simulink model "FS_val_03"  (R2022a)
settings: Solver=VariableStepAuto  StartTime=0.0  StopTime=300  RelTol=1e-3
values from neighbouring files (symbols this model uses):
  C = 6.3000e-04    (= 0.00063)    [maglev_init.m]
  g = 9.80    (= 9.8)    [maglev_init.m]
  K = 1.0e+03 * [-2.4567   -0.1235    0.0237]    [maglev_init.m]
  L1 = 0.6000    (= 0.6)    [maglev_init.m]
  m = 0.0300    (= 0.03)    [maglev_init.m]
  mpert = 0    [maglev_init.m]
  R = 45    [maglev_init.m]
  Ts = 0.005    [maglev_init.m]    (also in train_net.m)
  x1_0 = 0.1    [maglev_init.m]
  x1_d = 0.05    [maglev_init.m]
  x2_0 = 0    [maglev_init.m]
  x2_d = 0    [maglev_init.m]
  x3_0 = 0.2    [maglev_init.m]
undefined symbols (not defined in the file or in its folder): magnitude
libraries: fuzblock x1

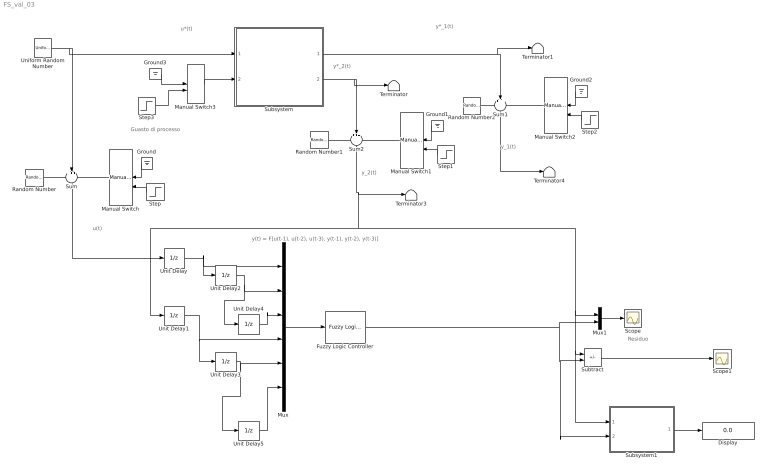
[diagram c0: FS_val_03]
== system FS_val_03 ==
  note: y(t) = F[u(t-1), u(t-2), u(t-3), y(t-1), y(t-2), y(t-3)]
  note: y_2(t)
  note: y*_1(t)
  note: u(t)
  note: y*_2(t)
  note: y_1(t)
  note: u*(t)
  note: Guasto di processo
  note: Residuo
  Display : Display
  Fuzzy Logic Controller : fuzblock/Fuzzy Logic  Controller  FIS=FIS03  OutputSampleNumber=101  DataType=double  FuzzifiedInputs=off  RuleFiringStrengths=off  RuleOutputs=off  AggregatedOutputs=off  SimulateUsing=Interpreted execution  OutOfRangeInputValueMessage=warning  NoRuleFiredMessage=warning  EmptyOutputFuzzySetMessage=warning
  Ground{,1..3} (4 alike) : Ground
  Manual Switch : ManualSwitch
  Manual Switch1 : ManualSwitch  CurrentSetting=0
  Manual Switch2 : ManualSwitch
  Manual Switch3 : ManualSwitch
  Mux : Mux  Inputs=6
  Mux1 : Mux  Inputs=2
  Random Number : RandomNumber  Variance=1e-9  Seed=1  SampleTime=Ts
  Random Number1 : RandomNumber  Variance=1e-6  Seed=3  SampleTime=Ts
  Random Number2 : RandomNumber  Variance=1e-9  Seed=2  SampleTime=Ts
  Scope : Scope
  Scope1 : Scope
  Step : Step  Time=150  SampleTime=0
  Step1 : Step  Time=150  SampleTime=0
  Step2 : Step  Time=150  SampleTime=0
  Step3 : Step  Time=15  After=2*R  SampleTime=0
  Subsystem : Subsystem
  Subsystem1 : Subsystem
  Subtract : Sum  Inputs=+-
  Sum : Sum  Inputs=+++
  Sum1 : Sum  Inputs=+++
  Sum2 : Sum  Inputs=+++
  Terminator{,1,3..4} (4 alike) : Terminator
  Uniform Random Number : UniformRandomNumber  Minimum=x1_d*0.9  Maximum=x1_d*1.1  Seed=1  SampleTime=0.5
  Unit Delay{,1..5} (6 alike) : UnitDelay  SampleTime=Ts  HasFrameUpgradeWarning=on
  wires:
  Subsystem/1(Out1) -> Terminator1/1, Sum1/2
  Subsystem/2(Out2) -> Terminator/1, Sum2/2
  Random Number/1 -> Sum/1
  Manual Switch/1 -> Sum/3
  Manual Switch2/1 -> Sum1/3
  Manual Switch1/1 -> Sum2/3
  Random Number1/1 -> Sum2/1
  Ground/1 -> Manual Switch/1
  Step/1 -> Manual Switch/2
  Ground1/1 -> Manual Switch1/1
  Step1/1 -> Manual Switch1/2
  Random Number2/1 -> Sum1/1
  Ground2/1 -> Manual Switch2/1
  Step2/1 -> Manual Switch2/2
  Manual Switch3/1 -> Subsystem/2(fs)
  Ground3/1 -> Manual Switch3/1
  Uniform Random Number/1 -> Subsystem/1(u), Sum/2
  Step3/1 -> Manual Switch3/2
  Sum/1 -> Unit Delay/1
  Unit Delay/1 -> Unit Delay2/1, Mux/1
  Unit Delay1/1 -> Mux/4, Unit Delay3/1
  Mux/1 -> Fuzzy Logic Controller/1
  Sum1/1 -> Terminator4/1
  Unit Delay2/1 -> Unit Delay4/1, Mux/2
  Unit Delay3/1 -> Unit Delay5/1, Mux/5
  Unit Delay4/1 -> Mux/3
  Unit Delay5/1 -> Mux/6
  Subtract/1 -> Scope1/1
  Subsystem1/1(VAF%) -> Display/1
  Mux1/1 -> Scope/1
  Fuzzy Logic Controller/1 -> Mux1/2, Subsystem1/2(y_prev), Subtract/2
  Sum2/1 -> Subsystem1/1(y_mis), Subtract/1, Mux1/1, Unit Delay1/1, Terminator3/1

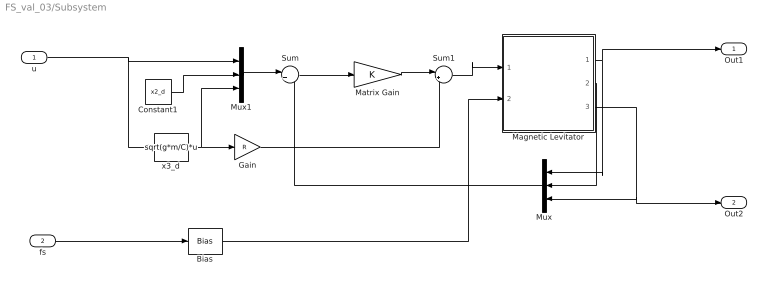
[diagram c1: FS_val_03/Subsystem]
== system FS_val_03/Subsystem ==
  u : Inport
  fs : Inport  Port=2
  Bias : Bias  Bias=R
  Constant1 : Constant  Value=x2_d
  Gain : Gain  Gain=R
  Magnetic Levitator : Subsystem  mask{m=m+mpert, R=R, L1=L1, C=C, g=g}
      mask prompts: m "ball's mass (m)"; R "Electromagnet's resistance (R)"; L1 "Electromagnet's inductance (L1)"; C "Magnetic force constant (C)"; g "Gravitational acceleration (g)"
  Matrix Gain : Gain  Gain=K  Multiplication=Matrix(K*u)  SaturateOnIntegerOverflow=on
  Mux : Mux  Inputs=3
  Mux1 : Mux  Inputs=3
  Sum : Sum  Inputs=|+-  InputSameDT=on  SaturateOnIntegerOverflow=on
  Sum1 : Sum  Inputs=|++  InputSameDT=on  SaturateOnIntegerOverflow=on
  x3_d : Fcn  Expr=sqrt(g*m/C)*u
  Out1 : Outport
  Out2 : Outport  Port=2
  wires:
  u/1 -> x3_d/1, Mux1/1
  Magnetic Levitator/2(x2) -> Mux/2
  x3_d/1 -> Mux1/3, Gain/1
  Mux1/1 -> Sum/1
  Gain/1 -> Sum1/2
  Mux/1 -> Sum/2
  Constant1/1 -> Mux1/2
  Sum/1 -> Matrix Gain/1
  Sum1/1 -> Magnetic Levitator/1(u)
  Magnetic Levitator/1(x1) -> Out1/1, Mux/1
  Magnetic Levitator/3(x3) -> Out2/1, Mux/3
  Matrix Gain/1 -> Sum1/1
  Bias/1 -> Magnetic Levitator/2(fs)
  fs/1 -> Bias/1

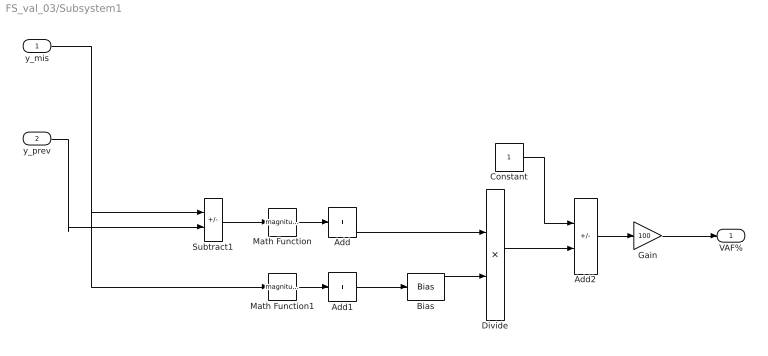
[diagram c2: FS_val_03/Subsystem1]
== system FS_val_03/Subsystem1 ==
  y_mis : Inport
  y_prev : Inport  Port=2
  Add : Sum  Inputs=+
  Add1 : Sum  Inputs=+
  Add2 : Sum  Inputs=+-
  Bias : Bias  Bias=1e-7
  Constant : Constant
  Divide : Product  Inputs=*/
  Gain : Gain  Gain=100
  Math Function : Math  Operator=magnitude^2
  Math Function1 : Math  Operator=magnitude^2
  Subtract1 : Sum  Inputs=+-
  VAF% : Outport
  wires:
  Add2/1 -> Gain/1
  Math Function/1 -> Add/1
  Bias/1 -> Divide/2
  y_mis/1 -> Math Function1/1, Subtract1/1
  Add1/1 -> Bias/1
  Math Function1/1 -> Add1/1
  Subtract1/1 -> Math Function/1
  Constant/1 -> Add2/1
  Divide/1 -> Add2/2
  Add/1 -> Divide/1
  y_prev/1 -> Subtract1/2
  Gain/1 -> VAF%/1

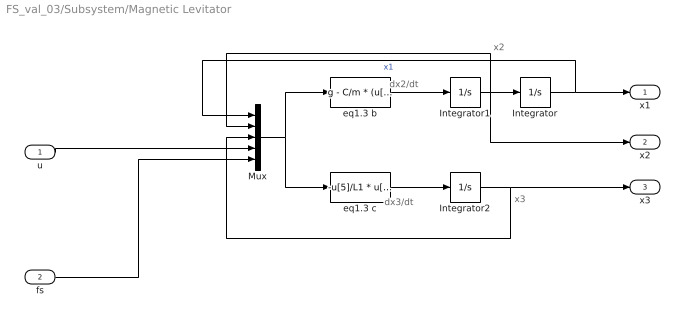
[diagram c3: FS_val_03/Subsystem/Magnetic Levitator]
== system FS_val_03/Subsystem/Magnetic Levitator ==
  note: x2
  note: x3
  note: dx2/dt
  note: dx3/dt
  u : Inport
  fs : Inport  Port=2
  Integrator : Integrator  InitialCondition=x1_0
  Integrator1 : Integrator  InitialCondition=x2_0
  Integrator2 : Integrator  InitialCondition=x3_0
  Mux : Mux  Inputs=5
  eq1.3 b : Fcn  Expr=g - C/m * (u[3] / u[1])^2
  eq1.3 c : Fcn  Expr=-u[5]/L1 * u[3] + (2*C)/L1 * ( u[2] * u[3] / u[1]^2 ) + 1/L1 * u[4]
  x1 : Outport
  x2 : Outport  Port=2
  x3 : Outport  Port=3
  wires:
  eq1.3 b/1 -> Integrator1/1
  Integrator1/1 -> Integrator/1, Mux/2, x2/1
  eq1.3 c/1 -> Integrator2/1
  Mux/1 -> eq1.3 b/1, eq1.3 c/1
  Integrator/1 -> Mux/1, x1/1  "x1"
  Integrator2/1 -> Mux/3, x3/1
  u/1 -> Mux/4
  fs/1 -> Mux/5
